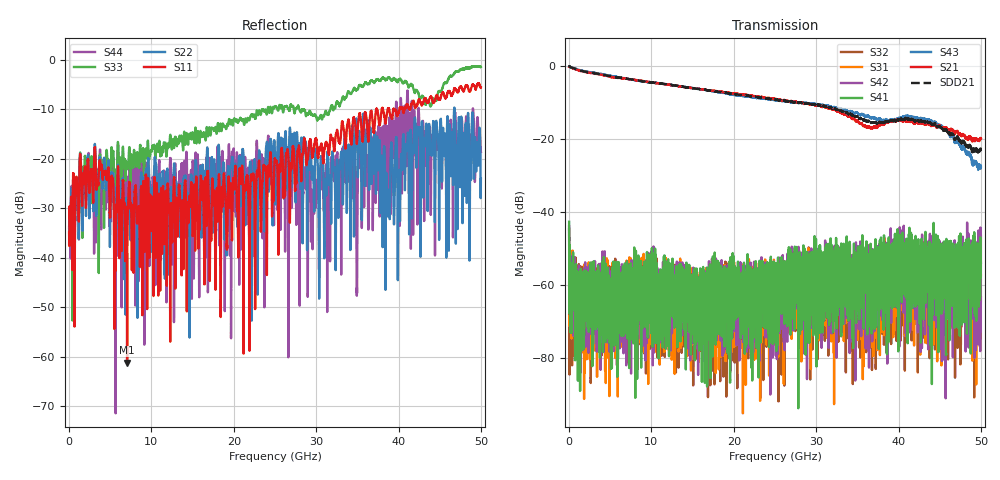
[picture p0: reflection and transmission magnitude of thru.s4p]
!Keysight Technologies,N5245A,MY49151038,A.10.65.06
!Date: Wednesday, June 07, 2023 10:56:02
!Correction: S11(Full 4 Port(1,2,3,4))
!S12(Full 4 Port(1,2,3,4))
!S13(Full 4 Port(1,2,3,4))
!S14(Full 4 Port(1,2,3,4))
!S21(Full 4 Port(1,2,3,4))
!S22(Full 4 Port(1,2,3,4))
!S23(Full 4 Port(1,2,3,4))
!S24(Full 4 Port(1,2,3,4))
!S31(Full 4 Port(1,2,3,4))
!S32(Full 4 Port(1,2,3,4))
!S33(Full 4 Port(1,2,3,4))
!S34(Full 4 Port(1,2,3,4))
!S41(Full 4 Port(1,2,3,4))
!S42(Full 4 Port(1,2,3,4))
!S43(Full 4 Port(1,2,3,4))
!S44(Full 4 Port(1,2,3,4))
!S4P File: Measurements: <S11,S12,S13,S14>,
!<S21,S22,S23,S24>,
!<S31,S32,S33,S34>,
!<S41,S42,S43,S44>:
# Hz S  RI  R 50
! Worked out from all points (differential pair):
!   5000 points, 10 MHz to 50 GHz, reference 50 ohm
!   strongest paths, dB at 10 MHz, 12.51 GHz, 25.01 GHz, 37.51 GHz, 50 GHz:
!     S21: -0.2, -5.3, -9.0, -16.5, -19.9
!     S43: -0.1, -5.2, -9.3, -14.7, -27.5
!     S41: -42.7, -68.5, -57.2, -54.6, -53.9
!     S42: -43.9, -56.2, -60.5, -63.0, -46.5
!     S31: -61.0, -66.4, -63.4, -57.6, -57.2
!     S32: -44.6, -63.7, -61.2, -53.1, -63.3
!   taken as a pair (ports 1,3 in; 2,4 out), SDD21 dB: -0.2, -5.2, -9.2, -15.6, -22.9
!   lowest |S11| = -61.2 dB at 7.05 GHz (marker M1), VSWR 1.00, Z = 50 - j0.0812 ohm
!   |S11| at or under -10 dB: start of sweep to 37.29 GHz; 38.12 GHz to 38.68 GHz (565 MHz wide, 1.47 % of centre); 39.46 GHz to 40.11 GHz (645.5 MHz wide, 1.62 % of centre)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
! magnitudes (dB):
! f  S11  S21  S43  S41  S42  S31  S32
! 10 MHz  -34.9  -0.2  -0.1  -42.7  -43.9  -61.0  -44.6
! 1.44 GHz  -21.0  -1.4  -1.2  -64.0  -76.7  -64.6  -62.8
! 7.05 GHz  -61.2  -3.5  -3.4  -58.8  -69.0  -56.5  -72.6
! 26.96 GHz  -21.0  -9.6  -9.9  -63.1  -61.6  -61.0  -56.6
! 38.64 GHz  -10.4  -15.5  -15.0  -64.6  -81.5  -59.0  -57.1
! 42.14 GHz  -9.1  -15.3  -14.2  -55.2  -52.0  -55.1  -59.4
! 50 GHz  -5.5  -19.9  -27.5  -53.9  -46.5  -57.2  -63.3
